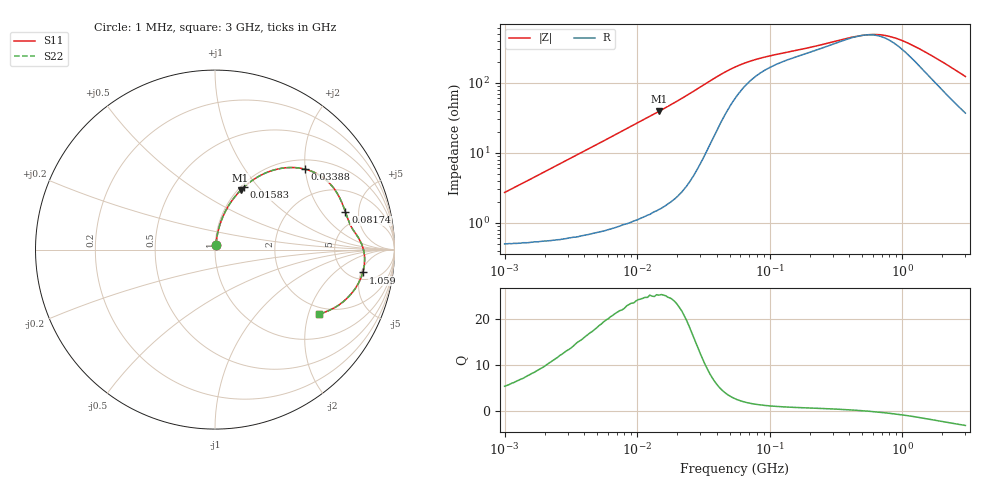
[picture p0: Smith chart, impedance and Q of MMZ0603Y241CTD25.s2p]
! S-parameter Generated by TDK Corporation
! Copyright(C) 2018 TDK Corporation.
! All Rights Reserved.
! TDK P/N: MMZ0603Y241CTD25 (Chip Bead)
! Property: |Z|=240¶ at 100MHz
! Size(LxWxT): 0.6x0.3x0.3mm, 0.024x0.012x0.012inches
! Model Type: s2p (Touchstone File Format Version 1.0)
! Frequency: DC=Yes Start=1MHz Stop=3000MHz 202points Log-sweep
! Model Generated on Aug. 6, 2018
! Port Assignments:
!  1 ---@@@--- 2
! Applicable Conditions:
!  Temperature = 25 degC
!  DC Bias Current = 0 A
!  Small Signal Operation
! Terms and conditions regarding TDK Simulation Models
! (1)This simulation model is being provided solely for informational purposes. Please refer to the specifications of the products in terms of detailed characteristics of such products.
! (2)In no event shall TDK Corporation of any of its subsidiaries be liable for any loss or damage arising, directly or indirectly,
!  From any information contained in this simulation model, including, but not limited to loss or damages arising from any inaccuracies, omissions or errors in connection with such information.
! (3)Any and all copyrights on this simulation model are owned by TDK Corporation.
!  Duplication or redistribution of this simulation model without prior written permission from TDK Corporation is prohibited.
! (4)This simulation model is subject to any modification or change without any prior notice.
! (5)Neither TDK Corporation nor any of its subsidiaries shall make any warranty, express or implied,
!  Including but not limited to the correctness, implied warranties of merchantability and fitness for a particular purpose with respect to this simulation models.
! (6)The use of this simulation model shall be deemed to have consented to the terms and conditions hereof.
# Hz S MA R 50
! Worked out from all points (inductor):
!   201 points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, 1 MHz to 3 GHz, reference 50 ohm
!   read as one part in series: L = 425 nH near 1.041 MHz
!   highest Q = 25.1 at 14.62 MHz (marker M1), where L = 425 nH
!   self-resonance near 511.8 MHz
!   S11 on the Smith chart (normalised r, x): 1 MHz: 1.01, +0.05; 15.83 MHz: 1.03, +0.85; 33.88 MHz: 1.22, +2.00; 81.74 MHz: 3.62, +3.54; 1.059 GHz: 6.46, -5.38; 3 GHz: 1.74, -2.35
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1000000  0.02703 77.9  0.9947 -1.5  0.9947 -1.5  0.02703 77.9
2055611  0.05459 81.1  0.9931 -3.1  0.9931 -3.1  0.05459 81.1
3900413  0.1024 80.5  0.9882 -5.9  0.9882 -5.9  0.1024 80.5
8686058  0.2222 74.7  0.9654 -12.8  0.9654 -12.8  0.2222 74.7
1.461624e7  0.3592 66.7  0.9191 -21.0  0.9191 -21.0  0.3592 66.7
1.583459e7  0.3858 65.0  0.9074 -22.7  0.9074 -22.7  0.3858 65.0
2.013356e7  0.4734 59.3  0.8606 -28.2  0.8606 -28.2  0.4734 59.3
2.459509e7  0.5538 53.3  0.8033 -33.6  0.8033 -33.6  0.5538 53.3
3.387922e7  0.6736 41.7  0.669 -42.0  0.669 -42.0  0.6736 41.7
4.307715e7  0.7285 32.5  0.5495 -45.4  0.5495 -45.4  0.7285 32.5
5.477226e7  0.7496 24.7  0.4468 -44.5  0.4468 -44.5  0.7496 24.7
8.173662e7  0.7564 16.0  0.3436 -37.4  0.3436 -37.4  0.7564 16.0
1.219755e8  0.7636 11.2  0.2911 -30.5  0.2911 -30.5  0.7636 11.2
2.136344e8  0.7855 6.9  0.2396 -23.2  0.2396 -23.2  0.7855 6.9
4.951867e8  0.8262 0.3  0.1739 -1.5  0.1739 -1.5  0.8262 0.3
6.296259e8  0.8331 -2.1  0.1703 10.4  0.1703 10.4  0.8331 -2.1
8.005644e8  0.8361 -4.9  0.1818 23.2  0.1818 23.2  0.8361 -4.9
1.059487e9  0.8333 -8.8  0.2175 35.8  0.2175 35.8  0.8333 -8.8
1.402151e9  0.8199 -13.5  0.279 43.4  0.279 43.4  0.8199 -13.5
1.855641e9  0.7905 -19.3  0.3637 45.8  0.3637 45.8  0.7905 -19.3
2.359433e9  0.7472 -25.2  0.4535 44.5  0.4535 44.5  0.7472 -25.2
3e9  0.6822 -31.9  0.5545 40.6  0.5545 40.6  0.6822 -31.9
